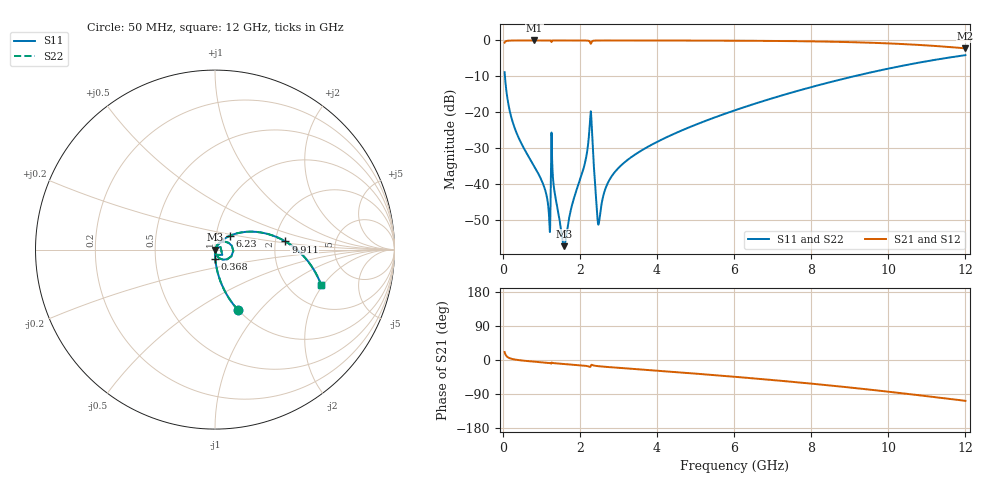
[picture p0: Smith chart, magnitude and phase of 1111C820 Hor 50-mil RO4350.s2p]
# GHz S MA R 50
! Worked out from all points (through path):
!   11951 points, 50 MHz to 12 GHz, reference 50 ohm
!   highest |S21| = -0.01 dB at 821 MHz (marker M1); lowest = -2.2 dB at 12 GHz (marker M2)
!   group delay of S21, straight-line fit = 24.9 ps
!   lowest |S11| = -57.4 dB at 1.591 GHz (marker M3), VSWR 1.00, Z = 50.1 - j0.0282 ohm
!   |S11| at or under -10 dB: 57.98 MHz to 9.113 GHz (9.055 GHz wide, 197 % of centre)
!   |S22| runs from -57.4 to -4.1 dB; largest |S21 - S12| = 0
!   S11 on the Smith chart (normalised r, x): 50 MHz: 1.00, -0.77; 368 MHz: 1.00, -0.10; 6.23 GHz: 1.17, +0.18; 9.911 GHz: 2.27, +0.25; 12 GHz: 2.98, -1.91
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0.05  0.3606 -69.1  0.9324 20.8  0.9324 20.8  0.3606 -69.1
0.188  0.1011 -85.2  0.9944 4.6  0.9944 4.6  0.1011 -85.2
0.368  0.04993 -88.8  0.998 0.4  0.998 0.4  0.04993 -88.8
0.821  0.01742 -91.2  0.9988 -4.4  0.9988 -4.4  0.01742 -91.2
1.075  0.009046 -89.3  0.9987 -6.6  0.9987 -6.6  0.009046 -89.3
1.185  0.004667 -80.0  0.9985 -7.6  0.9985 -7.6  0.004667 -80.0
1.308  0.01139 -88.8  0.998 -8.0  0.998 -8.0  0.01139 -88.8
1.591  0.001345 -12.1  0.9986 -10.5  0.9986 -10.5  0.001345 -12.1
2.042  0.01301 66.7  0.9977 -14.2  0.9977 -14.2  0.01301 66.7
2.283  0.1024 -3.9  0.8996 -16.3  0.8996 -16.3  0.1024 -3.9
2.326  0.03962 -71.0  0.978 -13.4  0.978 -13.4  0.03962 -71.0
2.438  0.004653 -60.5  0.9965 -15.9  0.9965 -15.9  0.004653 -60.5
2.498  0.002881 12.8  0.9973 -16.5  0.9973 -16.5  0.002881 12.8
2.663  0.008482 58.7  0.9978 -18.0  0.9978 -18.0  0.008482 58.7
2.891  0.01418 62.7  0.9979 -19.8  0.9979 -19.8  0.01418 62.7
4.034  0.03909 58.4  0.9968 -28.4  0.9968 -28.4  0.03909 58.4
6.025  0.106 44.0  0.9911 -44.4  0.9911 -44.4  0.106 44.0
6.23  0.1155 42.4  0.9899 -46.1  0.9899 -46.1  0.1155 42.4
8.017  0.2242 26.5  0.9701 -62.5  0.9701 -62.5  0.2242 26.5
9.911  0.3947 6.6  0.9129 -82.6  0.9129 -82.6  0.3947 6.6
10.009  0.4049 5.5  0.9084 -83.7  0.9084 -83.7  0.4049 5.5
12  0.6229 -18.4  0.7747 -107.7  0.7747 -107.7  0.6229 -18.4
